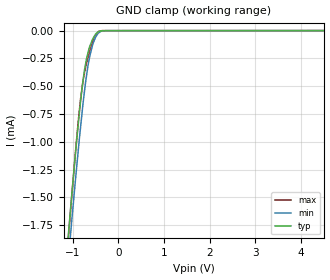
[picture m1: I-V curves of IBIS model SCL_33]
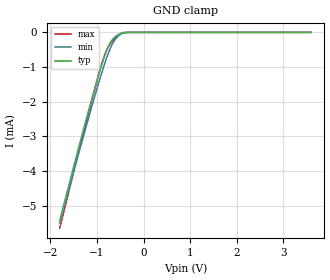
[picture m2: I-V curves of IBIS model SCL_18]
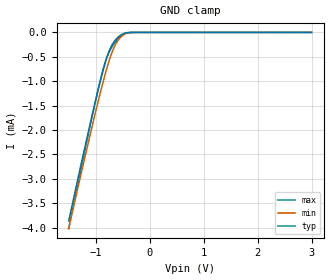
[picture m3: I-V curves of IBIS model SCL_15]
|Texas Instruments Incorporated
|Low-Power, Digital Temperature Sensor with Two-Wire Interface in WCSP
| Marketing part#   Digital Voltage Range   Package-type   #pins
|TMP103AYFFR   1.4 to 3.6   WCSP   4
|TMP103AYFFT   1.4 to 3.6   WCSP   4
|TMP103BYFFR   1.4 to 3.6   WCSP   4
|TMP103BYFFT   1.4 to 3.6   WCSP   4
|TMP103CYFFR   1.4 to 3.6   WCSP   4
|TMP103CYFFT   1.4 to 3.6   WCSP   4
|TMP103DYFFR   1.4 to 3.6   WCSP   4
|TMP103DYFFT   1.4 to 3.6   WCSP   4
|TMP103EYFFR   1.4 to 3.6   WCSP   4
|TMP103EYFFT   1.4 to 3.6   WCSP   4
|TMP103FYFFR   1.4 to 3.6   WCSP   4
|TMP103FYFFT   1.4 to 3.6   WCSP   4
|TMP103GYFFR   1.4 to 3.6   WCSP   4
|TMP103GYFFT   1.4 to 3.6   WCSP   4
|TMP103HYFFR   1.4 to 3.6   WCSP   4
|TMP103HYFFT   1.4 to 3.6   WCSP   4
[IBIS Ver]   4.0
[File name]   tmp103.ibs
|   SIMDE V2.0 201002
[File Rev]   1.0
[Date]   02/10/2011
[Source]   Texas Instruments Incorporated.
   Analog-eLab, HPA
   12500 TI Blvd
   Dallas, TX -75243
   For Support e-mail: elab_ibis@list.ti.com
[Notes]   Revision History:
   1.0: 02/10/2011
   - Initial version of the model
   - Initial Model generated from simulations in TISPICED
   - Model names with a trailing _33 contains the model for
   3.3V (3.0V and 3.6V).
   - Model names with trailing _18 contains
   the model for 1.8V (1.62V and 1.98V) operation.
   - Model names with trailing _15 contains the model for 1.5V
   (1.4V and 1.6V)operation.
   - Model not matched to measurements
   - C_comp although listed in numerical order of value are
   obtained from varying PVT conditions. For PVT conditions
   for each specific value refer the buffer description under
   respective [Model]. IBIS model user is responsible for using
   appropriate C_comp to simulate for Signal Integrity.
[Disclaimer]
 This product is designed as an aid for customers of Texas Instruments.
 No warranties, either expressed or implied, with respect to this third
 party software (if any) or with respect to its fitness for any
 particular purpose is claimed by Texas Instruments or the author. The
 software (if any) is provided solely on an "as is" basis. The entire
 risk as to its quality and performance is with the customer
[Copyright] (C) Copyright 2011 Texas Instruments Incorporated.
   All rights reserved.
|   TMP103
[Component]   tmp103yff
[Manufacturer] TI
[Package]   |4 pin YFF - WCSP package
| variable   typ   min   max
R_pkg   4.95000E-02   3.60000E-02   6.30000E-02
L_pkg   2.78500E-01nH  2.64000E-01nH   2.93000E-01nH
C_pkg   5.52000E-01pF  3.98000E-01pF   7.06000E-01pF
[Pin] signal_name  model_name  R_pin  L_pin C_pin
A1   VP   POWER   0.106   0.701nH   0.623pf
A2   GND   GND   0.128   0.661nH   0.526pf
B1   SDA   SDA   0.036   0.264nH   0.398pf
B2   SCL   SCL   0.063   0.293nH   0.706pf
|   Model Selectors
[Model Selector]  SCL
SCL_33   3.3V digital input
SCL_18   1.8V digital input
SCL_15   1.5V digital input
|NOTES   Model SCL split into two Models SCL_33, SCL_18, and SCL_15
|   to accomodate vast voltage range of 1.4 to 3.6V
|   SCL_33 operates in voltage range of 3.0 - 3.3 - 3.6
|   SCL_18 operates in voltage range of 1.92 - 1.8 - 1.98
|   SCL_15  operates in voltage range of 1.4 -.1.5 - 1.6
|   The max pin frequency for Model SCL is 3.4MHz
|   This is referenced with SCL pin in datasheet
[Model Selector]  SDA
SDA_33  3.3V digital I/O open drain
SDA_18  1.8V digital I/O open drain
SDA_15  1.5V digital I/O open drain
| Models and submodels in the file (6): SCL_33 (Input), SCL_18 (Input), SCL_15 (Input), SDA_33 (I/O_open_drain), SDA_18 (I/O_open_drain), SDA_15 (I/O_open_drain)
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|NOTES   Model SDA split into two Models SDA_33, SDA_18, and SDA_15
|   to accomodate vast voltage range of 1.4 to 3.6V
|   SDA_33 operates in voltage range of 3.0 - 3.3 - 3.6
|   SDA_18 operates in voltage range of 1.92 - 1.8 - 1.98
|   SDA_14  operates in voltage range of 1.4 -.1.5 - 1.6
|   The max pin frequency for Model SDA is 3.4MHz
|   This is referenced with SDA pin in datasheet
|   SCL_33   3.3V digital input Model
[Model] SCL_33
Model_type   Input
| Signals   SCL(1)
Vinl = 0.99
Vinh = 2.31
|   typ   min   max
|   (nom PVT)   (Fast PVT)   (slow PVT)
|Average
C_comp   5.4900360e-13  5.4418680e-13  5.5891860e-13
| Where   nom PVT is  Nominal Process, 3.3V, 27C
|   Fast PVT is Strong Process, 3.6V, -40C
|   Slow PVT is Weak Process, 3.0V, 125C
[Voltage Range]   3.3   3   3.6
[Temperature Range]   27   125   -40
|Ambient Temperature   27   125   -40
[Power Clamp Reference]   3.3   3   3.6
[GND Clamp Reference]   0   0   0
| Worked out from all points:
|   GND clamp passes 1 mA (typ) near -0.91 V on its own axis
[GND Clamp]
|   Voltage   I(typ)   I(min)   I(max)
-3.3V     -13.46mA   -13.1mA    -14.03mA
-1.087V   -1.801mA   -2.021mA   -1.829mA
-1.028V   -1.517mA   -1.747mA   -1.528mA
-938.5mV  -1.107mA   -1.342mA   -1.09mA
-840.7mV  -690.3uA   -922.9uA   -666.5uA
-746.4mV  -369.8uA   -564.8uA   -390.9uA
-669.3mV  -208.8uA   -328.8uA   -249.3uA
-622.2mV  -138.7uA   -224.4uA   -178.2uA
-550.1mV  -68.18uA   -112.6uA   -90.26uA
-431.8mV  -7.715uA   -20.4uA    -8.3uA
-283mV    -626.1nA   -693.1nA   -641.4nA
6.6V      0A         0A         0A
[POWER Clamp]
|   SCR cell for ESD function. Effects occurr above VDD x 2
|   Voltage   I(typ)   I(min)   I(max)
-3.3V     0A         0A         0A
0V        0A         0A         0A
6.6V      0A         0A         0A
|   SCL_18   1.8V digital input Model
[Model] SCL_18
Model_type   Input
| Signals   SCL(1)
Vinl = 0.54
Vinh = 1.26
|   typ   min   max
|   (nom PVT)   (Fast PVT)   (slow PVT)
|Average
C_comp   5.8962220e-13  5.6768840e-13  5.9923480e-13
| Where   nom PVT is  Nominal Process, 1.8V, 27C
|   Fast PVT is Strong Process, 1.98V, -40C
|   Slow PVT is Weak Process, 1.62V, 125C
[Voltage Range]   1.8   1.62   1.98
[Temperature Range]   27   125   -40
|Ambient Temperature   27   125   -40
[Power Clamp Reference]   1.8   1.62   1.98
[GND Clamp Reference]   0   0   0
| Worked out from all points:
|   GND clamp passes 1 mA (typ) near -0.91 V on its own axis
[GND Clamp]
|   Voltage   I(typ)   I(min)   I(max)
-1.8V     -5.422mA   -5.502mA   -5.649mA
-1.266V   -2.675mA   -2.874mA   -2.767mA
-1.017V   -1.467mA   -1.695mA   -1.473mA
-894.6mV  -913.6uA   -1.15mA    -888.4uA
-816.7mV  -598.5uA   -825.2uA   -581.8uA
-750.5mV  -381uA     -577.7uA   -399.9uA
-714.6mV  -291.5uA   -458.9uA   -325.4uA
-648.4mV  -174uA     -278.8uA   -215.6uA
-544mV    -62.85uA   -107.4uA   -83.2uA
-426.2mV  -7.015uA   -17.92uA   -7.862uA
-287.6mV  -738.1nA   -782.2nA   -427nA
3.595V    0A         0A         0A
[POWER Clamp]
|   SCR cell for ESD function. Effects occurr above VDD x 2
|   Voltage   I(typ)   I(min)   I(max)
-1.8V     0A         0A         0A
0V        0A         0A         0A
3.6V      0A         0A         0A
|   SCL_15   1.8V digital input Model
[Model] SCL_15
Model_type   Input
| Signals   SCL(1)
Vinl = 0.45
Vinh = 1.05
|   typ   min   max
|   (nom PVT)   (Fast PVT)   (slow PVT)
|Average
C_comp   5.9438280e-13  5.8018180e-13  6.0447370e-13
| Where   nom PVT is  Nominal Process, 1.5V, 27C
|   Fast PVT is Strong Process, 1.6V, -40C
|   Slow PVT is Weak Process, 1.4V, 125C
[Voltage Range]   1.5   1.4   1.6
[Temperature Range]   27   125   -40
|Ambient Temperature   27   125   -40
[Power Clamp Reference]   1.5   1.4   1.6
[GND Clamp Reference]   0   0   0
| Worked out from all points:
|   GND clamp passes 1 mA (typ) near -0.91 V on its own axis
[GND Clamp]
|   Voltage   I(typ)   I(min)   I(max)
-1.5V     -3.861mA   -4.014mA   -4.019mA
-1.278V   -2.733mA   -2.928mA   -2.827mA
-1.073V   -1.733mA   -1.956mA   -1.758mA
-944.8mV  -1.135mA   -1.37mA    -1.12mA
-859.1mV  -764.8uA   -999uA     -737.7uA
-792.7mV  -514uA     -731.9uA   -507.7uA
-712.5mV  -286.9uA   -452.2uA   -321.2uA
-624.9mV  -142.6uA   -229.6uA   -181.8uA
-516.2mV  -42.52uA   -76.66uA   -56.11uA
-413.8mV  -5.086uA   -14.06uA   -7.981uA
-283.3mV  -720.1nA   -701.7nA   -385nA
2.995V    0A         0A         0A
[POWER Clamp]
|   SCR cell for ESD function. Effects occurr above VDD x 2
|   Voltage   I(typ)   I(min)   I(max)
-1.5V     0A         0A         0A
0V        0A         0A         0A
3V        0A         0A         0A
